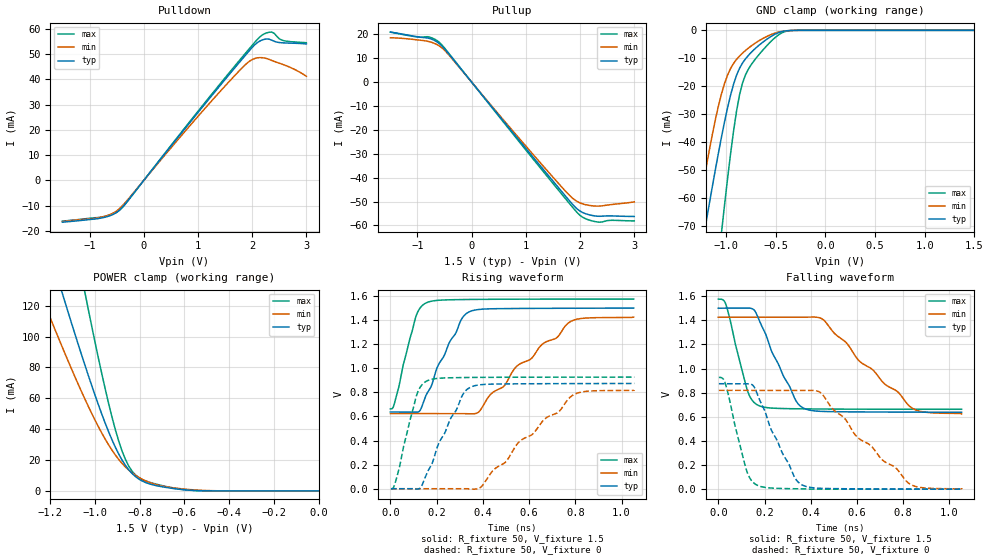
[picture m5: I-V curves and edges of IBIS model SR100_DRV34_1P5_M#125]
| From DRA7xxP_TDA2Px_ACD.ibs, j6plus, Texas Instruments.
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| Model based on original model for DDR_SEIOPB_V
|   Sub model SR100_DRV34_1P5
[model]   SR100_DRV34_1P5_M#125
|[Description]  [1.5V-I/O-X-X]
|   , ,
|[Input Load]
|[Output Drive]
|Voltage   1.5V
|Mode   I/O
Model_type   I/O
Polarity   Non-Inverting
Enable   Active-Low
Vinl =  0.65
Vinh =  0.85
Cref =  15.0000pF
Rref =  100.0000M
Vref =  0V
Vmeas =  0.75
C_comp   2p   2p   2p
[Model Spec]
Vinl   0.65   0.6125   0.6875
Vinh   0.85   0.8125   0.8875
[Receiver Thresholds]
Tslew_ac = 0.5n
Vth = 0.75
Vth_max = 0.7875
Vth_min = 0.675
Vinh_ac = 0.175
Vinh_dc = 0.1
Vinl_ac = -0.175
Vinl_dc = -0.1
[Temperature Range]   25   125   -40
[Voltage Range]   1.5   1.425   1.575
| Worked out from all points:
|   slope of the pulldown table from 0 to 0.225 V, typ, clamps not added: 36.8 ohm
|   slope of the pullup table from 0 to 0.225 V, typ, clamps not added: 35.8 ohm
|   GND clamp passes 1 mA (typ) near -0.48 V on its own axis
|   POWER clamp passes 1 mA (typ) near -0.62 V on its own axis
|   rising waveform, R_fixture 50, V_fixture 1.5: 20-80 % time 126ps typ, 292ps min, 68.2ps max; typ from 0.637 V to 1.5 V
|   rising waveform, R_fixture 50, V_fixture 0: 20-80 % time 124ps typ, 285ps min, 68.1ps max; typ from 0 V to 0.874 V
|   falling waveform, R_fixture 50, V_fixture 1.5: 20-80 % time 123ps typ, 269ps min, 69.3ps max; typ from 1.5 V to 0.637 V
|   falling waveform, R_fixture 50, V_fixture 0: 20-80 % time 124ps typ, 274ps min, 69.1ps max; typ from 0.874 V to 0 V
[POWER_clamp]
-1.5V     302.8mA    223.9mA    484.4mA
-1.242V   174.3mA    127.3mA    279.1mA
-1.136V   123.3mA    89.68mA    196.8mA
-1.045V   81.65mA    59.62mA    128.8mA
-1.03V    75mA       54.92mA    117.8mA
-939.4mV  38.44mA    29.91mA    56.84mA
-893.9mV  23.93mA    20.41mA    32.31mA
-848.5mV  13.61mA    13.43mA    15.91mA
-803mV    7.623mA    8.663mA    8.564mA
-712.1mV  3.022mA    3.561mA    3.877mA
-575.8mV  470.5uA    872uA      449uA
0V        112.6nA    435.6nA    613.8nA
[Pulldown]
-1.5V     -16.54mA   -16.32mA   -16.11mA
-727.3mV  -14.62mA   -14.26mA   -14.29mA
-545.5mV  -13.24mA   -12.72mA   -13.05mA
-409.1mV  -10.94mA   -10.36mA   -11.07mA
1.227V    32.84mA    30.87mA    33.41mA
1.818V    48.09mA    44.61mA    48.84mA
2V        52.62mA    47.82mA    53.46mA
2.182V    55.55mA    48.58mA    57.5mA
2.273V    55.99mA    48.2mA     58.42mA
2.364V    55.5mA     47.46mA    58.71mA
2.545V    54.48mA    46.06mA    55.55mA
3V        54mA       41.23mA    54.49mA
[Pullup]
-1.5V     20.96mA    18.6mA     20.95mA
-1V       19mA       17.69mA    18.93mA
-772.7mV  18.26mA    16.89mA    18.84mA
-590.9mV  16.04mA    15.07mA    16.54mA
-409.1mV  11.43mA    11.07mA    11.7mA
1.409V    -38.97mA   -37.46mA   -39.88mA
1.773V    -48.83mA   -46.66mA   -49.96mA
1.909V    -52.33mA   -49.44mA   -53.68mA
2.045V    -54.57mA   -50.97mA   -56.55mA
2.273V    -56.03mA   -51.89mA   -58.38mA
2.591V    -56.03mA   -51.23mA   -57.86mA
3V        -56.26mA   -50.14mA   -58.12mA
[GND_clamp]
-1.5V     -133.6mA   -115.7mA   -234.3mA
-1.288V   -87.29mA   -67.59mA   -156.8mA
-1.197V   -68.11mA   -48.64mA   -124.4mA
-1.045V   -38.25mA   -22.77mA   -72.51mA
-1.015V   -32.88mA   -19.1mA    -62.74mA
-954.5mV  -23.3mA    -13.72mA   -44.4mA
-863.6mV  -13.6mA    -9.192mA   -23.11mA
-803mV    -10.18mA   -7.193mA   -15.89mA
-681.8mV  -5.771mA   -4.027mA   -9.287mA
-500mV    -1.264mA   -914.7uA   -2.429mA
-348.5mV  -52.39uA   -75.11uA   -85.87uA
1.5V      112.6nA    528.1nA    514.5nA
[Ramp]
dV/dt_f 0.51823631/0.12330659n 0.48142319/0.26932586n 0.54806259/69.321081p
dV/dt_r  0.5262361/0.12477107n  0.4935804/0.28678756n 0.55783658/68.304787p
R_load = 50
[Rising Waveform]
R_fixture = 50
V_fixture = 1.5
V_fixture_min = 1.425
V_fixture_max = 1.575
0s        637.3mV    624.3mV    663.1mV
17.43ps   637.1mV    624.2mV    707.7mV
110.4ps   635.1mV    624.2mV    1.43V
155.8ps   781.8mV    624.2mV    1.544V
305.6ps   1.4V       624.1mV    1.571V
344.4ps   1.472V     621.8mV    1.572V
382.8ps   1.489V     638.8mV    1.572V
544.6ps   1.497V     1.013V     1.574V
777.2ps   1.499V     1.386V     1.575V
1.053ns   1.5V       1.425V     1.575V
[Rising Waveform]
R_fixture = 50
V_fixture = 0
V_fixture_min = 0
V_fixture_max = 0
2.529ps   0V         0V         0V
35.1ps    0V         0V         147mV
114.2ps   -2.955mV   0V         780.8mV
160.7ps   140.9mV    0V         897.6mV
310.1ps   770.9mV    0V         923.2mV
350.9ps   846.8mV    -3.198mV   924.1mV
391.9ps   863.9mV    14.11mV    924.7mV
556.1ps   871.3mV    387.2mV    926.1mV
789.7ps   873.1mV    777mV      926.6mV
1.055ns   874.1mV    819mV      926.7mV
[Falling Waveform]
R_fixture = 50
V_fixture = 1.5
V_fixture_min = 1.425
V_fixture_max = 1.575
0s        1.5V       1.425V     1.575V
31.83ps   1.5V       1.425V     1.536V
125.8ps   1.501V     1.425V     818.4mV
174.1ps   1.412V     1.425V     693.7mV
332.4ps   745.1mV    1.425V     666.3mV
372.6ps   668.1mV    1.425V     665.4mV
455.5ps   644mV      1.403V     664.1mV
609.4ps   640.2mV    1.064V     662.9mV
838.3ps   638.4mV    672.1mV    662.4mV
1.053ns   637.3mV    624.3mV    662.3mV
[Falling Waveform]
R_fixture = 50
V_fixture = 0
V_fixture_min = 0
V_fixture_max = 0
2.529ps   874.1mV    819mV      926.7mV
32.2ps    874.3mV    819.1mV    865.4mV
125.1ps   874.5mV    819.1mV    139.2mV
170.9ps   775.9mV    819mV      30.39mV
278.9ps   292.6mV    819mV      5.364mV
367.5ps   30.29mV    819.2mV    2.495mV
445ps     6.924mV    795.6mV    0V
598.2ps   2.646mV    436.9mV    0V
828.5ps   0V         42.88mV    0V
1.055ns   0V         0V         0V
